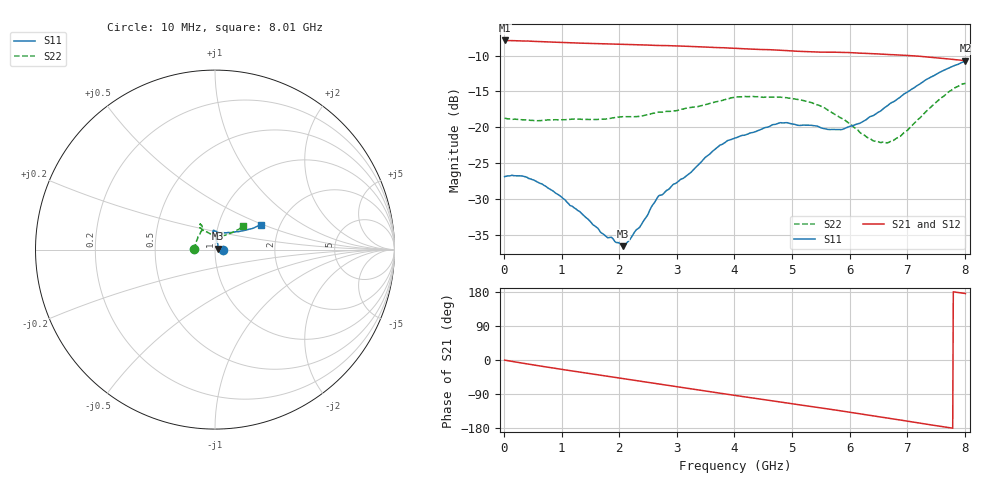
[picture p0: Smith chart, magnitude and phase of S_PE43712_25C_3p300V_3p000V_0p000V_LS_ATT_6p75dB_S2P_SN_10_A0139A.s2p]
! DEVICE ID: PE43712
! File Path: z:\PE43713\PE43713_CHAR_NOM_04292014\AMB\3p300\LS_ATT_6p75dB\PE43713_AMB_3p300V_3p000V_0p000V_LS_ATT_6p75dB_S2P_SN_10_A0139A.s2p
! Serial: 10
! Lot: A0139A
! Temp: 25C
! VDD: 3.300
! VSS: 0.000
! Control_Hi: 3.000
! Control_Lo: 0.000
! Attenuation Step: 6.75dB
! Port 1: RF1
! Port 2: RF2
! ThroughPath:1-2
! IDD: 0.0001471468
! ISS: -1.021e-007
#  Hz  S  RI  R  50
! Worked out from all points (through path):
!   801 points, 10 MHz to 8.01 GHz, reference 50 ohm
!   highest |S21| = -7.89 dB at 10 MHz (marker M1); lowest = -10.7 dB at 8.01 GHz (marker M2)
!   group delay of S21, straight-line fit = 63.3 ps
!   lowest |S11| = -36.6 dB at 2.07 GHz (marker M3), VSWR 1.03, Z = 51.4 + j0.511 ohm
!   |S11| at or under -10 dB: start of sweep to end of sweep
!   |S22| runs from -22.2 to -13.9 dB; largest |S21 - S12| = 0.0013
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1e7  0.0453 -6.28e-05  0.4033 -0.0023  0.4032 -0.00223  -0.1157 0.000725
3.3e8  0.0449 -0.00798  0.3953 -0.0596  0.395 -0.0591  -0.1123 0.0109
6.3e8  0.0388 -0.012  0.3807 -0.1085  0.3808 -0.1086  -0.1094 0.0201
9.6e8  0.0309 -0.0127  0.358 -0.1577  0.3582 -0.1578  -0.1086 0.0306
1.35e9  0.0229 -0.00999  0.325 -0.2087  0.325 -0.2087  -0.1053 0.0428
1.71e9  0.0178 -0.00346  0.2891 -0.2504  0.2891 -0.2504  -0.0988 0.0562
2.07e9  0.0139 0.00496  0.2481 -0.2867  0.2482 -0.2866  -0.0952 0.0706
2.37e9  0.0142 0.0148  0.2101 -0.3119  0.21 -0.3118  -0.0859 0.0829
2.68e9  0.0163 0.0287  0.1689 -0.3316  0.1689 -0.3316  -0.0769 0.1019
3.23e9  0.00892 0.047  0.0904 -0.3549  0.0904 -0.355  -0.0726 0.1163
3.72e9  0.00412 0.0733  0.0201 -0.359  0.0199 -0.3589  -0.0737 0.1328
4.01e9  -0.00141 0.0842  -0.0212 -0.3551  -0.0212 -0.355  -0.0809 0.1403
4.79e9  -0.00957 0.1072  -0.1226 -0.3219  -0.1226 -0.3222  -0.0882 0.1363
5.35e9  0.00155 0.1028  -0.1837 -0.2818  -0.1837 -0.2816  -0.0843 0.1218
5.63e9  0.0135 0.0956  -0.2107 -0.2592  -0.2106 -0.2593  -0.0697 0.1109
5.88e9  0.0273 0.0929  -0.2354 -0.2355  -0.2349 -0.2356  -0.0525 0.1018
6.18e9  0.0516 0.0934  -0.2589 -0.2027  -0.2584 -0.2028  -0.0271 0.0878
6.39e9  0.0726 0.0953  -0.2728 -0.1787  -0.2723 -0.1785  -0.00878 0.081
6.68e9  0.1059 0.0973  -0.2882 -0.1427  -0.2879 -0.1428  0.0214 0.0756
6.99e9  0.1411 0.103  -0.3 -0.103  -0.2996 -0.1029  0.0514 0.079
7.7e9  0.2244 0.1248  -0.3001 -0.0112  -0.2998 -0.0115  0.132 0.1138
8.01e9  0.2538 0.1383  -0.2908 0.023  -0.2902 0.0226  0.156 0.1296
